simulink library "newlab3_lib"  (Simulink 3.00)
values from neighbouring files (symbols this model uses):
  h = 0.05    [initlab3.m]
undefined symbols (not defined in the file or in its folder): AIno, AOno, R, S, T
libraries: cstblocks x1

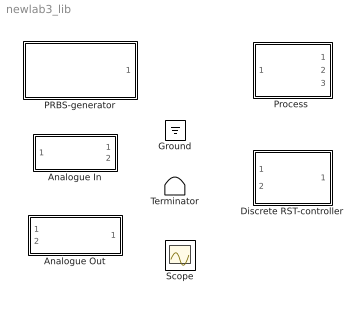
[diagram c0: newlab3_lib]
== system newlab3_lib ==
  Analogue In : Subsystem  mask(AnalogueIOBlock){h=h, AIno=AIno}
      mask prompts: h "Sample period"; AIno "Input port number"
      mask help: Analogue input block for use on PC running Linux.
  Analogue Out : Subsystem  mask(AnalogueIOBlock){h=h, AOno=AOno}
      mask prompts: h "Sample period"; AOno "Output port number"
      mask help: Analogue output block for use on PC running Linux
  Discrete RST-controller : Subsystem  mask(ControllerMaskBlock){R=R, S=S, T=T, h=h}
      mask prompts: R "R-polynomial"; S "S-polynomial"; T "T-polynomial"; h "Sample period"
      mask help: Discrete RST-controller (forward shift) R(q)u = -S(q)y + T(q)y_ref
  Ground : Ground
  PRBS-generator : Subsystem  mask(PRBSblockMask){h=h, N=5, Amp=2, offset=0, seed=0}
      mask prompts: h "Sample time (h)"; N "PRBS period (N)"; Amp "Amplitude"; seed "Random seed"
      mask help: A (P)RBS-generator
  "Process " : Subsystem  mask(SIMO Process){AOu=0, AIy=0, AIu=1, h=h}
      mask prompts: AOu "AO  u"; AIy "AI y"; AIu "AI u"; h "Sample Period"
      mask help: Process communication block. For use with Linux on PC with I/O.
  Scope : Scope
  Terminator : Terminator

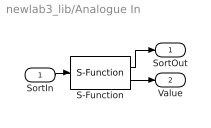
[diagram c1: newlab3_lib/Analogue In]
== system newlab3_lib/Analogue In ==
  SortIn : Inport  Port=1  PortWidth=-1  SampleTime=-1  DataType=auto
  S-Function : S-Function  FunctionName=analogin  Parameters=h AIno  PortCounts=[]  SFunctionModules=''
  SortOut : Outport  Port=1  InitialOutput=0
  Value : Outport  Port=2  InitialOutput=0
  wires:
  S-Function/2 -> Value/1
  SortIn/1 -> S-Function/1
  S-Function/1 -> SortOut/1

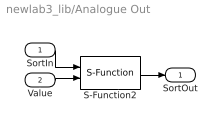
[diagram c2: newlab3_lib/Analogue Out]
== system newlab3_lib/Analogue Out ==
  SortIn : Inport  Port=1  PortWidth=-1  SampleTime=-1  DataType=auto
  Value : Inport  Port=2  PortWidth=-1  SampleTime=-1  DataType=auto
  S-Function2 : S-Function  FunctionName=analogout  Parameters=h AOno  PortCounts=[]  SFunctionModules=''
  SortOut : Outport  Port=1  InitialOutput=0
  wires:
  Value/1 -> S-Function2/2
  S-Function2/1 -> SortOut/1
  SortIn/1 -> S-Function2/1

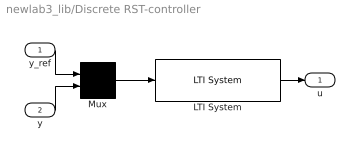
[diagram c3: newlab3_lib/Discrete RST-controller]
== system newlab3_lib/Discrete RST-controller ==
  y_ref : Inport  Port=1  PortWidth=-1  SampleTime=-1  DataType=auto
  y : Inport  Port=2  PortWidth=-1  SampleTime=-1  DataType=auto
  LTI System : cstblocks/LTI System  sys=ss(tf({T, -S},{R,R},h))  IC=[0]
  Mux : Mux  Inputs=2
  u : Outport  Port=1  InitialOutput=0
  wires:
  y/1 -> Mux/2
  LTI System/1 -> u/1
  y_ref/1 -> Mux/1
  Mux/1 -> LTI System/1

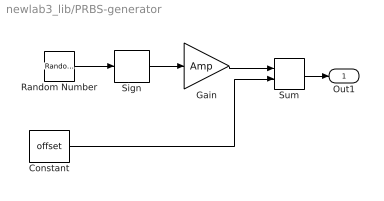
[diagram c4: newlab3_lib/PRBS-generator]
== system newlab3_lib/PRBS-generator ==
  Constant : Constant  Value=offset
  Gain : Gain  Gain=Amp  SaturateOnIntegerOverflow=on
  Random Number : RandomNumber  Mean=0  Variance=1  Seed=seed  SampleTime=h*N
  Sign : Signum
  Sum : Sum  Inputs=++  SaturateOnIntegerOverflow=on
  Out1 : Outport  Port=1  InitialOutput=0
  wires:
  Random Number/1 -> Sign/1
  Sign/1 -> Gain/1
  Gain/1 -> Sum/1
  Constant/1 -> Sum/2
  Sum/1 -> Out1/1

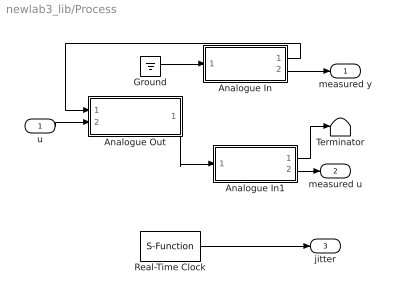
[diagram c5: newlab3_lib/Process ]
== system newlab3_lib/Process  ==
  u : Inport  Port=1  PortWidth=-1  SampleTime=-1  DataType=auto
  Analogue In : Subsystem  mask(AnalogueIOBlock){h=h, AIy=AIy}
      mask prompts: h "Sample period"; AIy "Input port number"
      mask help: Analogue input block for use on PC running Linux.
  Analogue In1 : Subsystem  mask(AnalogueIOBlock){h=h, AIu=AIu}
      mask prompts: h "Sample period"; AIu "Input port number"
      mask help: Analogue input block for use on PC running Linux.
  Analogue Out : Subsystem  mask(AnalogueIOBlock){h=h, AOu=AOu}
      mask prompts: h "Sample period"; AOu "Output port number"
      mask help: Analogue output block for use on PC running Linux
  Ground : Ground
  Real-Time Clock : S-Function  FunctionName=timer  Parameters=h  PortCounts=[]  SFunctionModules=''
  Terminator : Terminator
  measured y : Outport  Port=1
  measured u : Outport  Port=2
  jitter : Outport  Port=3
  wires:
  Analogue In/1(SortOut) -> Analogue Out/1(SortIn)
  u/1 -> Analogue Out/2(Value)
  Real-Time Clock/1 -> jitter/1
  Analogue In/2(Value) -> measured y/1
  Ground/1 -> Analogue In/1(SortIn)
  Analogue In1/1(SortOut) -> Terminator/1
  Analogue In1/2(Value) -> measured u/1
  Analogue Out/1(SortOut) -> Analogue In1/1(SortIn)

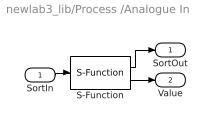
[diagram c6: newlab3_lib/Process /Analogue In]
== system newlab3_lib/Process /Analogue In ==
  SortIn : Inport  Port=1  PortWidth=-1  SampleTime=-1  DataType=auto
  S-Function : S-Function  FunctionName=analogin  Parameters=h AIy  PortCounts=[]  SFunctionModules=''
  SortOut : Outport  Port=1  InitialOutput=0
  Value : Outport  Port=2  InitialOutput=0
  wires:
  S-Function/1 -> SortOut/1
  SortIn/1 -> S-Function/1
  S-Function/2 -> Value/1

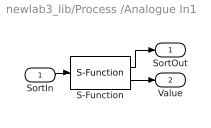
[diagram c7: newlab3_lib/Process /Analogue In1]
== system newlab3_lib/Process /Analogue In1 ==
  SortIn : Inport  Port=1  PortWidth=-1  SampleTime=-1  DataType=auto
  S-Function : S-Function  FunctionName=analogin  Parameters=h AIu  PortCounts=[]  SFunctionModules=''
  SortOut : Outport  Port=1  InitialOutput=0
  Value : Outport  Port=2  InitialOutput=0
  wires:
  S-Function/2 -> Value/1
  SortIn/1 -> S-Function/1
  S-Function/1 -> SortOut/1

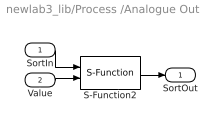
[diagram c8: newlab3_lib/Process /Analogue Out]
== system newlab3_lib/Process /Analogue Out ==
  SortIn : Inport  Port=1  PortWidth=-1  SampleTime=-1  DataType=auto
  Value : Inport  Port=2  PortWidth=-1  SampleTime=-1  DataType=auto
  S-Function2 : S-Function  FunctionName=analogout  Parameters=h AOu  PortCounts=[]  SFunctionModules=''
  SortOut : Outport  Port=1  InitialOutput=0
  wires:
  SortIn/1 -> S-Function2/1
  S-Function2/1 -> SortOut/1
  Value/1 -> S-Function2/2
